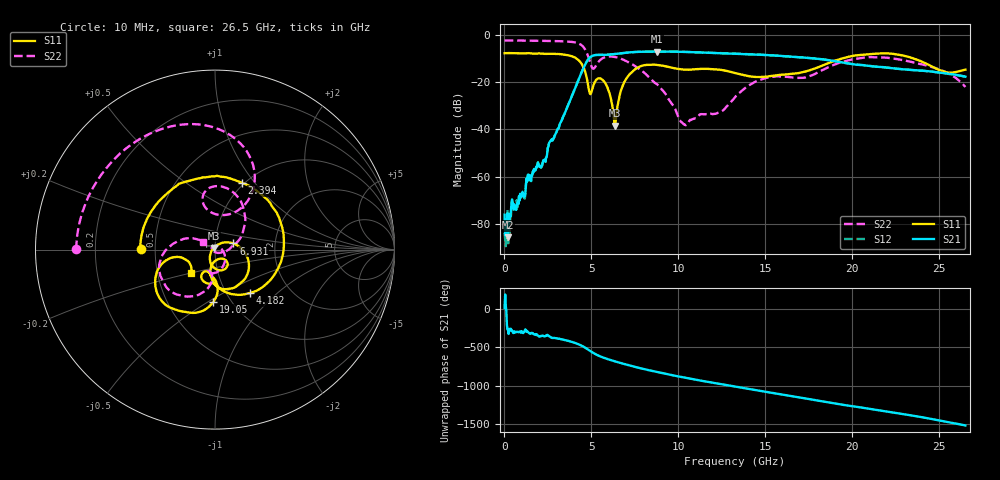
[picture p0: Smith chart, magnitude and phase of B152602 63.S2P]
!  2-Port S-parameters saved by WinCal
! VAR MeasName=S-Parameters (CALIBRATED_DATA) read from VNA (N5242A)
! VAR MeasDate=2016-1-5 16:34:43
! VAR NAME=B152602 63
! VAR FILENAME=B152602 63.S2P
! VAR DATE=2016-1-5 16:34:43
! VAR PHYS_PORTS=1,2
# Hz S DB R 50
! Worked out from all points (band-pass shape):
!   801 points, 10 MHz to 26.5 GHz, reference 50 ohm
!   highest |S21| = -6.94 dB at 8.785 GHz (marker M1); lowest = -85.8 dB at 208.7 MHz (marker M2)
!   |S21| within 3 dB of the highest: 4.854 GHz to 17.87 GHz (13.02 GHz wide, 115 % of centre)
!   lowest |S11| = -38.4 dB at 6.368 GHz (marker M3), VSWR 1.02, Z = 49.3 + j0.94 ohm
!   |S11| at or under -10 dB: 4.156 GHz to 19.37 GHz (15.21 GHz wide, 129 % of centre); 23.57 GHz to end of sweep
!   |S22| runs from -38.2 to -2.2 dB; largest |S21 - S12| = 0.0029
!   S11 on the Smith chart (normalised r, x): 10 MHz: 0.41, +0.00; 2.394 GHz: 0.98, +0.87; 4.182 GHz: 1.28, -0.69; 6.931 GHz: 1.22, +0.09; 19.05 GHz: 0.83, -0.53; 26.5 GHz: 0.74, -0.20
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1e7  -7.64 179.6  -76.14 8.8  -83.80 -49.2  -2.24 179.9
2.08675e8  -7.61 170.8  -85.76 96.7  -89.37 163.2  -2.25 176.8
1.367612e9  -7.58 118.6  -59.09 53.8  -59.92 58.4  -2.33 158.7
2.3941e9  -7.92 67.9  -51.96 11.8  -51.76 10.8  -2.44 141.2
3.387475e9  -8.21 9.5  -34.33 -43.4  -34.30 -43.5  -2.61 119.4
4.182175e9  -10.14 -51.0  -20.31 -95.6  -20.31 -95.6  -3.31 91.3
4.447075e9  -12.29 -76.4  -15.56 -122.4  -15.54 -122.4  -4.33 76.4
4.91065e9  -24.77 -80.2  -9.49 172.8  -9.49 172.9  -11.20 57.6
5.109325e9  -21.43 -44.4  -8.62 144.4  -8.61 144.4  -14.23 83.2
5.738462e9  -19.74 -91.6  -8.37 79.4  -8.35 79.5  -9.43 97.5
6.3676e9  -38.42 127.3  -8.01 33.9  -8.00 33.9  -9.27 76.6
6.930512e9  -19.35 18.6  -7.52 -2.2  -7.51 -2.1  -10.74 58.1
8.784812e9  -12.66 -69.2  -6.94 -104.3  -6.91 -104.2  -20.87 7.7
8.851038e9  -12.72 -71.1  -6.94 -107.6  -6.91 -107.6  -21.36 4.6
1.037421e10  -14.62 -93.2  -7.10 -177.4  -7.09 -177.4  -37.91 -115.8
1.186428e10  -14.35 -105.9  -7.53 121.0  -7.48 120.9  -33.31 115.2
1.3255e10  -16.05 -118.0  -7.85 66.8  -7.83 66.6  -26.32 -14.6
1.520864e10  -17.42 -103.2  -8.48 -8.2  -8.48 -8.2  -17.87 -86.8
1.769208e10  -14.52 -87.2  -9.79 -103.0  -9.76 -102.8  -16.99 -97.1
1.904969e10  -10.70 -91.8  -11.09 -155.2  -11.03 -155.1  -12.26 -104.9
2.209604e10  -7.76 -139.5  -13.87 98.2  -13.81 97.8  -9.65 -160.8
2.65e10  -14.60 -136.4  -17.60 -78.7  -17.59 -78.8  -22.00 146.6
